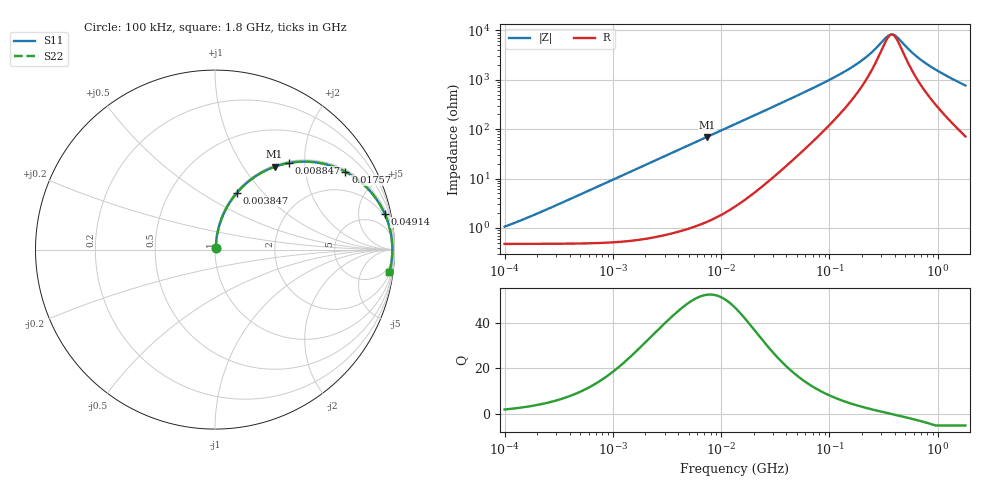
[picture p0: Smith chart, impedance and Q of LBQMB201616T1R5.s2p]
! LBQMB201616T1R5  S-PARAMETER MODEL  ( General Type )
! Model Generated by TAIYO YUDEN Corporation (http://www.ty-top.com)
! Version 1.0
! TAIYO YUDEN Control No. 191025NI43SB-FBB
! Copyright(c) 2019 TAIYO YUDEN CO.,LTD. All Rights Reserved.
! Product Description (link to TY-COMPAS)
! https://ds.yuden.co.jp/TYCOMPAS/or/detail?pn=LBQMB201616T1R5J&u=M
! Products Name : Inductors
! Characteristics :
!  Inductance : 1.5 uH , SRF(min) : 135 MHz , DC Resistance(max) : 0.611 Ohm , Rated Current : 350 mA
!  Case Size : 2.0 x 1.6 / 0.079 x 0.063 [mm/inch] , Thickness : 1.6 / 0.063 [mm/inch]
!  (Conditions: Temperature = 25 degC , DC Bias Current/Voltage = 0A / 0V)
! External Node Assignments :
!  1  o---GGG---o  2
! GND o---------o GND
! Frequency Range : 0.1MHz  -  1800MHz  [ 402 STEP ]
# MHz S RI R 50
! Freq[MHz].  S11 Real  S11 Imag  S21 Real  S21 Imag  S12 Real  S12 Imag  S22 Real  S22 Imag
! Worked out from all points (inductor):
!   401 points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, 100 kHz to 1.8 GHz, reference 50 ohm
!   read as one part in series: L = 1.51 uH near 151.7 kHz
!   highest Q = 52.4 at 7.453 MHz (marker M1), where L = 1.49 uH
!   self-resonance near 376.3 MHz
!   S11 on the Smith chart (normalised r, x): 100 kHz: 1.01, +0.02; 3.847 MHz: 1.02, +0.72; 8.847 MHz: 1.03, +1.66; 17.57 MHz: 1.08, +3.30; 49.14 MHz: 1.54, +9.34; 1.8 GHz: 2, -15
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0.1  0.0048 0.00939  0.9952 -0.00939  0.9952 -0.00939  0.0048 0.00939
0.516129  0.00716 0.0483  0.9928 -0.0483  0.9928 -0.0483  0.00716 0.0483
1.277529  0.0194 0.1178  0.9806 -0.1178  0.9806 -0.1178  0.0194 0.1178
2.66389  0.0649 0.2333  0.9351 -0.2333  0.9351 -0.2333  0.0649 0.2333
3.846706  0.1214 0.3155  0.8786 -0.3155  0.8786 -0.3155  0.1214 0.3155
5.420303  0.2108 0.398  0.7892 -0.398  0.7892 -0.398  0.2108 0.398
7.452807  0.3318 0.4614  0.6682 -0.4614  0.6682 -0.4614  0.3318 0.4614
8.84682  0.4099 0.4823  0.5901 -0.4823  0.5901 -0.4823  0.4099 0.4823
13.41641  0.611 0.4769  0.389 -0.4769  0.389 -0.4769  0.611 0.4769
17.56533  0.7263 0.4337  0.2737 -0.4337  0.2737 -0.4337  0.7263 0.4337
27.97575  0.8656 0.3241  0.1344 -0.3241  0.1344 -0.3241  0.8656 0.3241
49.1428  0.9457 0.1994  0.0543 -0.1994  0.0543 -0.1994  0.9457 0.1994
69.24595  0.967 0.1422  0.033 -0.1422  0.033 -0.1422  0.967 0.1422
121.6389  0.9821 0.0762  0.0179 -0.0762  0.0179 -0.0762  0.9821 0.0762
184.4683  0.9862 0.0428  0.0138 -0.0428  0.0138 -0.0428  0.9862 0.0428
241.5136  0.9874 0.0254  0.0126 -0.0254  0.0126 -0.0254  0.9874 0.0254
357.3983  0.9881 0.00286  0.0119 -0.00286  0.0119 -0.00286  0.9881 0.00286
384.6512  0.9881 -0.00122  0.0119 0.00122  0.0119 0.00122  0.9881 -0.00122
413.9822  0.9881 -0.00529  0.0119 0.00529  0.0119 0.00529  0.9881 -0.00529
597.7978  0.9874 -0.0265  0.0126 0.0265  0.0126 0.0265  0.9874 -0.0265
821.96  0.9858 -0.0477  0.0142 0.0477  0.0142 0.0477  0.9858 -0.0477
1800  0.9721 -0.1246  0.0279 0.1246  0.0279 0.1246  0.9721 -0.1246
